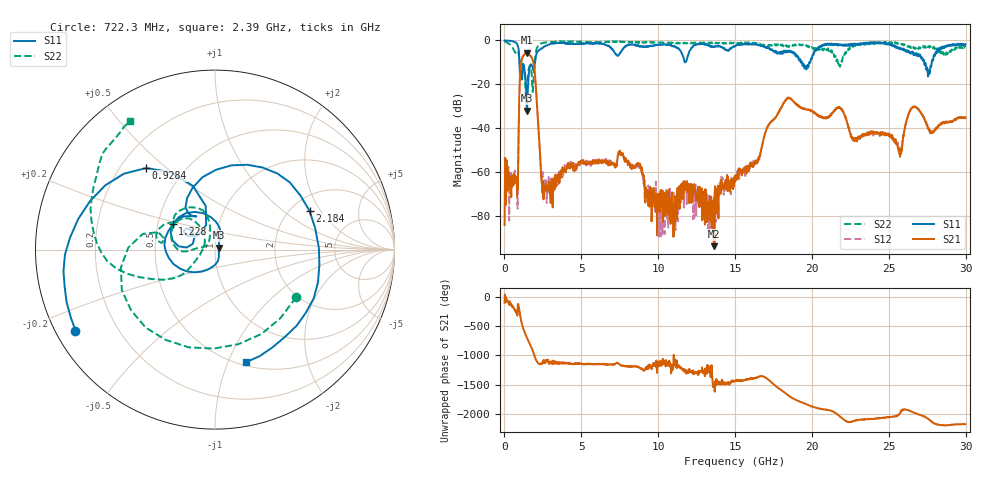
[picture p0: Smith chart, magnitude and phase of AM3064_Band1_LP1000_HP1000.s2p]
# Hz S DB R 50.0
!freq dBS11 angS11 dBS21 angS21 dBS12 angS12 dBS22 angS22
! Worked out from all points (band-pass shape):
!   1600 points, 10 MHz to 29.98 GHz, reference 50 ohm
!   highest |S21| = -5.66 dB at 1.435 GHz (marker M1); lowest = -93.9 dB at 13.62 GHz (marker M2)
!   |S21| within 3 dB of the highest: 1.128 GHz to 1.83 GHz (702.1 MHz wide, 47.5 % of centre)
!   lowest |S11| = -32.1 dB at 1.453 GHz (marker M3), VSWR 1.05, Z = 52.2 + j1.19 ohm
!   |S11| at or under -10 dB: 973.7 MHz to 1.992 GHz (1.018 GHz wide, 68.7 % of centre); 19.36 GHz to 19.83 GHz (476.7 MHz wide, 2.43 % of centre); 27.3 GHz to 27.79 GHz (494.3 MHz wide, 1.79 % of centre)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
!   |S22| runs from -25.9 to -0.4 dB; largest |S21 - S12| = 0.0076
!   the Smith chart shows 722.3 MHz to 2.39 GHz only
!   S11 on the Smith chart (normalised r, x): 722.3 MHz: 0.06, -0.27; 928.4 MHz: 0.31, +0.43; 1.228 GHz: 0.60, +0.18; 2.184 GHz: 2.51, +1.59; 2.39 GHz: 0.53, -1.16
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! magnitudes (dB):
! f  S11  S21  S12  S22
! 10 MHz  0.0  -84.2  -53.5  -0.4
! 722.3 MHz  -0.9  -64.6  -64.1  -5.6
! 928.4 MHz  -4.5  -39.4  -39.5  -6.3
! 1.228 GHz  -11.2  -7.1  -7.0  -10.9
! 1.435 GHz  -26.9  -5.7  -5.6  -23.3
! 1.453 GHz  -32.1  -5.7  -5.6  -21.4
! 1.884 GHz  -13.4  -10.1  -10.1  -18.3
! 2.184 GHz  -4.9  -36.8  -36.9  -2.5
! 2.39 GHz  -3.7  -62.2  -62.1  -1.3
! 2.99 GHz  -1.6  -72.1  -66.3  -0.8
! 5.015 GHz  -1.4  -55.8  -55.4  -0.6
! 7.545 GHz  -5.6  -52.3  -51.5  -0.7
! 10 GHz  -2.0  -70.1  -76.0  -0.9
! 13.62 GHz  -2.7  -93.9  -78.4  -1.1
! 15 GHz  -2.5  -64.5  -62.5  -1.4
! 18.34 GHz  -5.5  -26.9  -26.7  -2.4
! 19.99 GHz  -8.3  -32.4  -32.3  -3.2
! 25 GHz  -1.4  -43.0  -42.8  -1.0
! 25.75 GHz  -3.4  -51.2  -52.1  -1.5
! 26.63 GHz  -6.8  -30.4  -30.2  -3.2
! 27.56 GHz  -16.3  -39.9  -40.2  -2.7
! 29.98 GHz  -1.8  -35.4  -35.2  -3.1
